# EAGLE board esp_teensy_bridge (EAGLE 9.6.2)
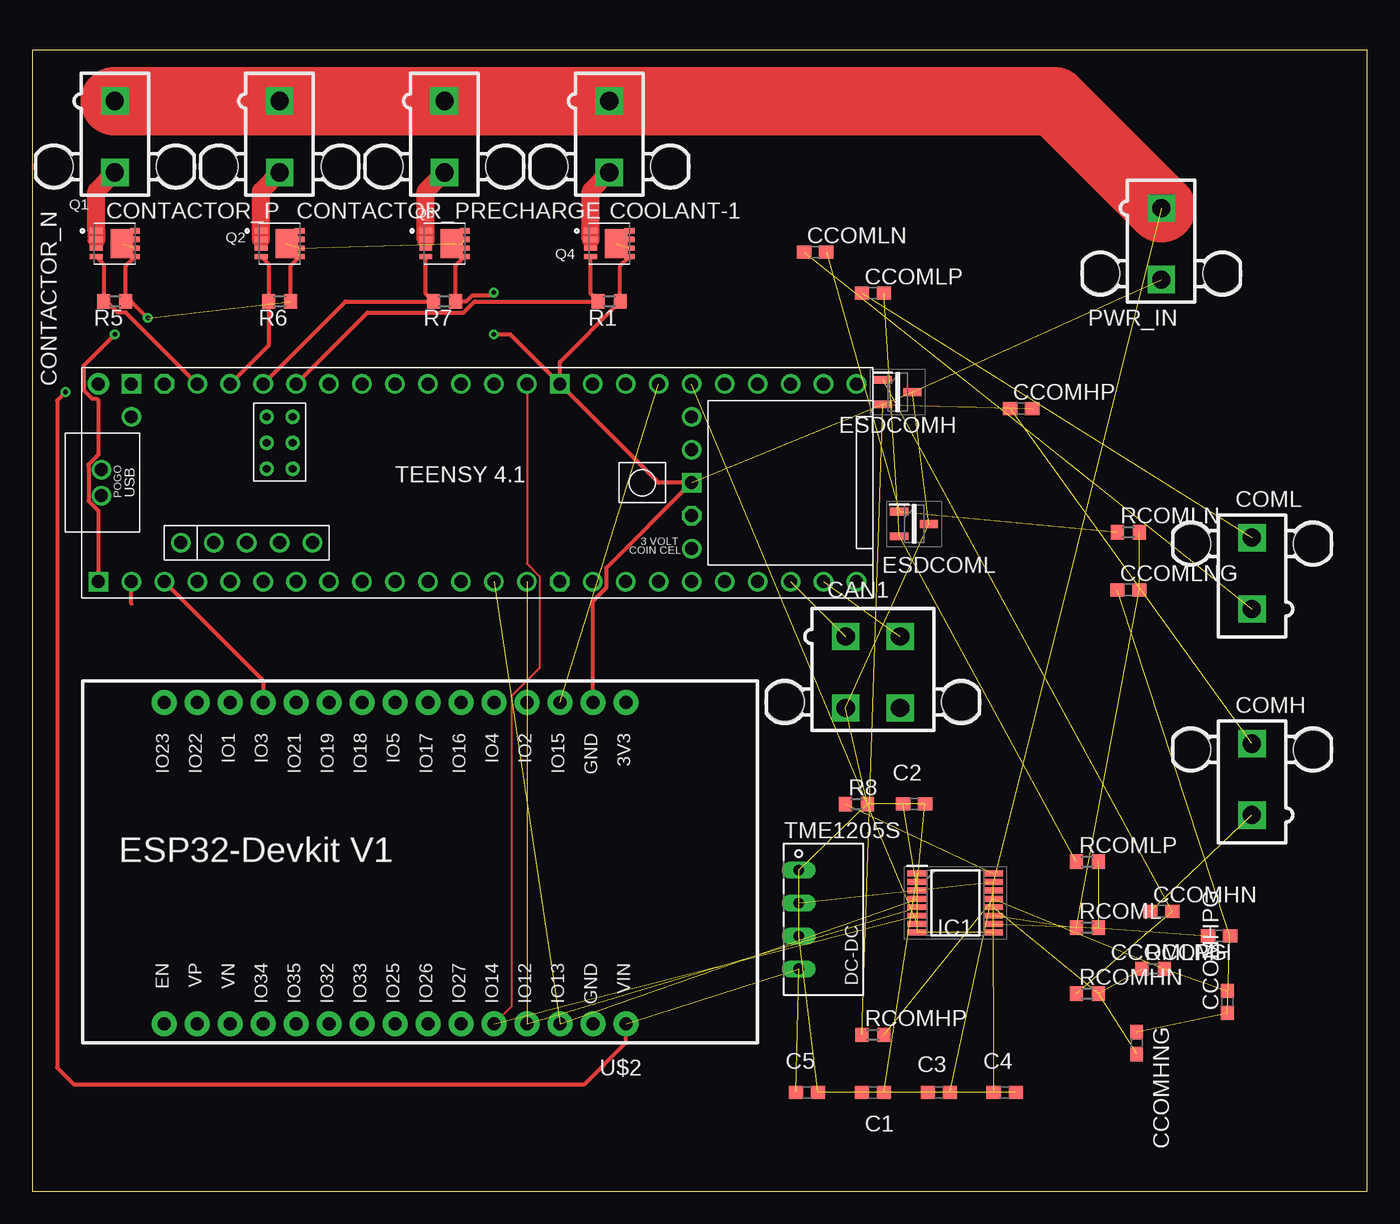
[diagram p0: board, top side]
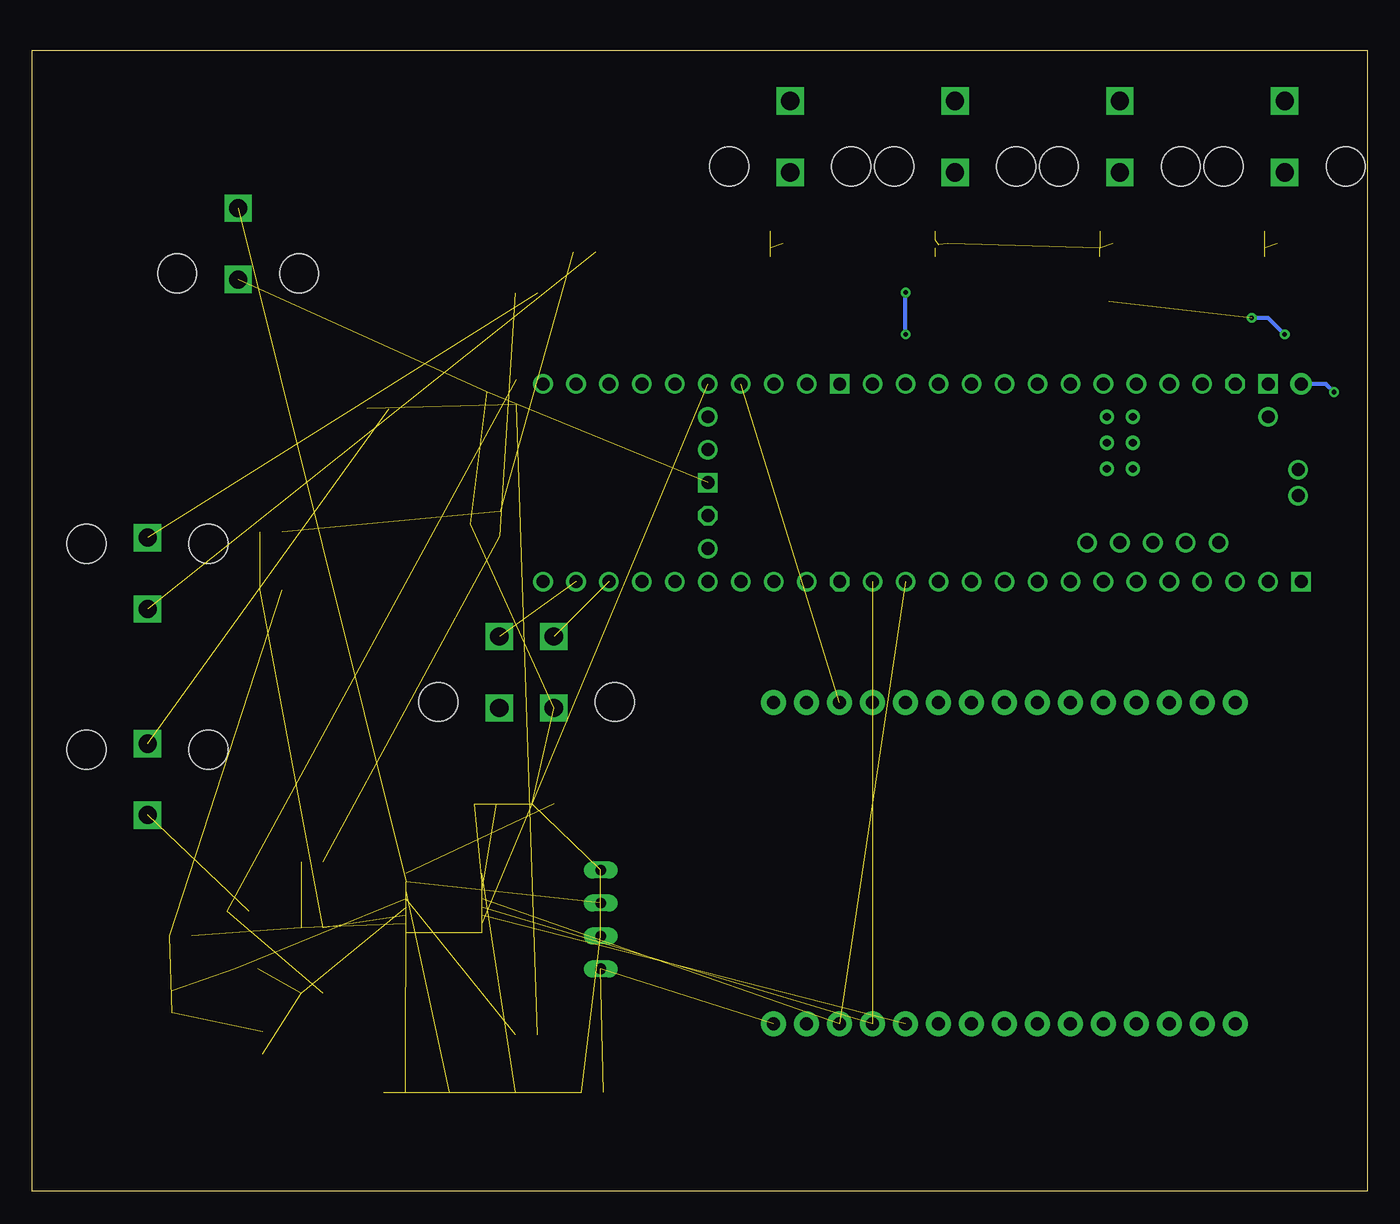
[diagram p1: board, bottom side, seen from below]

Size 102.85 x 87.94 mm. Coordinates in mm from the lower left corner, seen from the top.
Outline: 0,0 102.85,0 102.85,87.94 0,87.94 0,0
Copper layers (1*16): Top 0.035mm / dielectric 1.5mm / Bottom 0.035mm
Design rules "default": minimum track width 6mil, minimum drill 0.35mm, track to track 6mil, track to pad 6mil, pad to pad 6mil, via to via 6mil, smd to smd 6mil, copper to edge 40mil, drill to drill 6mil, minimum pad ring 10mil, minimum via ring 8mil, stop-mask expansion 4mil, vias tented up to drill 0mil, thermal gap 10mil

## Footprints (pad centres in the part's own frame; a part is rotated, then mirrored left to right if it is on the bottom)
C0603 = smd 1.1 x 1: 1 -0.85,0; 2 0.85,0
5566-4 = drill 1.4 square: 1 2.1,-2.75; 2 -2.1,-2.75; 3 2.1,2.75; 4 -2.1,2.75 | hole 3: 6.8,2.29; -6.8,2.29
5566-2 = drill 1.4 square: 1 0,-2.75; 2 0,2.75 | hole 3: 4.7,2.29; -4.7,2.29
SOT95P255X150-3N = smd 1.4 x 0.6: 1 -1.15,0.95; 2 -1.15,-0.95; 3 1.15,0
SOP65P640X120-16N = smd 1.475 x 0.45: 1 -2.938,2.275; 2 -2.938,1.625; 3 -2.938,0.975; 4 -2.938,0.325; 5 -2.938,-0.325; 6 -2.938,-0.975; 7 -2.938,-1.625; 8 -2.938,-2.275; 9 2.938,-2.275; 10 2.938,-1.625; 11 2.938,-0.975; 12 2.938,-0.325; 13 2.938,0.325; 14 2.938,0.975; 15 2.938,1.625; 16 2.938,2.275
VISHAY_SIS468DN-T1-GE3 = smd 0.99 x 0.405: 1 -1.435,0.99; 2 -1.435,0.33; 3 -1.435,-0.33; 4 -1.435,-0.99 | smd 0.76 x 0.405: 5 1.55,-0.99; 6 1.55,-0.33; 7 1.55,0.33; 8 1.55,0.99 | smd 1.725 x 2.235: 9 0.557,0
R0603 = smd 1 x 1.1: 1 -0.85,0; 2 0.85,0
NME = drill 0.813 long: 1 0,3.81; 2 0,1.27; 3 0,-1.27; 4 0,-3.81
ESP32-DEVKITV1 = drill 1 pad 1.93: 1 -22.87,-13.54; 2 -20.33,-13.54; 3 -17.79,-13.54; 4 -15.25,-13.54; 5 -12.71,-13.54; 6 -10.17,-13.54; 7 -7.63,-13.54; 8 -5.09,-13.54; 9 -2.55,-13.54; 10 -0.01,-13.54; 11 2.53,-13.54; 12 5.07,-13.54; 13 7.61,-13.54; 14 10.15,-13.54; 15 12.69,-13.54; 16 12.69,11.23; 17 10.15,11.23; 18 7.61,11.23; 19 5.07,11.23; 20 2.53,11.23; 21 -0.01,11.23; 22 -2.55,11.23; 23 -5.09,11.23; 24 -7.63,11.23; 25 -10.17,11.23; 26 -12.71,11.23; 27 -15.25,11.23; 28 -17.79,11.23; 29 -20.33,11.23; 30 -22.87,11.23
TEENSY41 = drill 1: 0-RX1/CS1/CRX2 -27.94,-7.62; 1-TX1/MISO1/CTX2 -25.4,-7.62; 2-OUT2 -22.86,-7.62; 3-LRCLK2 -20.32,-7.62; 4-BCLK2 -17.78,-7.62; 5-IN2 -15.24,-7.62; 6-OUT1D -12.7,-7.62; 7-RX2/OUT1A -10.16,-7.62; 8-TX2/IN1 -7.62,-7.62; 9-OUT1C -5.08,-7.62; 10-CS\MQSR -2.54,-7.62; 11-MOSI/CTX1 0,-7.62; 12-MISO/MQSL 2.54,-7.62; 13-SCK/LED 2.54,7.62; 14-A0/TX3/SPDIF_OUT 0,7.62; 15-A1/RX3/SPDIF_IN -2.54,7.62; 16-A2/RX4/SCL1 -5.08,7.62; 17-A3/TX4/SDA1 -7.62,7.62; 18-A4/SDA0 -10.16,7.62; 19-A5/SCL0 -12.7,7.62; 20-A6/TX5/LRCLK1 -15.24,7.62; 21-A7/RX5/BCLK1 -17.78,7.62; 22-A8/CTX1 -20.32,7.62; 23-A9/CRX1/MCLK1 -22.86,7.62; 24-A10/TX6/SCL2 7.62,-7.62; 25-A11/RX6/SDA2 10.16,-7.62; 26-A12/MOSI1 12.7,-7.62; 27-A13/SCK1 15.24,-7.62; 28-RX7 17.78,-7.62; 29-TX7 20.32,-7.62; 30-CRX3 22.86,-7.62; 31-CTX3 25.4,-7.62; 32-OUT1B 27.94,-7.62; 33-MCLK2 27.94,7.62; 34-RX8 25.4,7.62; 35-TX8 22.86,7.62; 36-PWM 20.32,7.62; 37-PWM 17.78,7.62; 38-A14/CS/IN1 15.24,7.62; 39-A15/CS/OUT1A 12.7,7.62; 40-A16/CS1 10.16,7.62; 41-A17/MISO1 7.62,7.62; +5V -24.13,-4.62; D+ -30.25,-1; D- -30.25,1; DM -21.59,-4.62; DP -19.05,-4.62; GND4 -16.51,-4.62; GND5 -13.97,-4.62; ON/OFF 15.24,5.08; PROGRAM 15.24,2.54; VBAT 15.24,-5.08; VUSB -27.94,5.08 | drill 1 octagon: 3V3-1 5.08,-7.62; 3V3-2 15.24,-2.54; 3V3-3 -25.4,7.62 | drill 0.6: G -15.51,3.08; LED -17.51,3.08; R+ -17.51,5.08; R- -15.51,5.08; T+ -15.51,1.08; T- -17.51,1.08 | drill 1 square: GND1 -30.48,-7.62; GND2 15.24,0; GND3 5.08,7.62; GND6 -27.94,7.62 | drill 1 pad 1.676: VIN -30.48,7.62

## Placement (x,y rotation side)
C1  0.22μF  [C0603]  64.77,7.62 180 top
C2  0.1μF  [C0603]  67.94,29.84 0 top
C3  0.22uF  [C0603]  69.85,7.62 0 top
C4  0.1μF  [C0603]  74.93,7.62 0 top
C5  0.22μF  [C0603]  59.69,7.62 0 top
CAN1  5566-4  [5566-4]  64.77,40.01 180 top
CCOMHN  2.2nf  [C0603]  87,21.59 0 top
CCOMHNG  220 pF  [C0603]  85.09,11.43 270 top
CCOMHP  2.2nf  [C0603]  76.2,60.33 0 top
CCOMHPG  220 pF  [C0603]  92.08,14.61 90 top
CCOMLN  2.2nf  [C0603]  60.33,72.39 0 top
CCOMLNG  220 pF  [C0603]  84.45,46.36 0 top
CCOMLP  2.2nf  [C0603]  64.77,69.22 0 top
CCOMLPG  220 pF  [C0603]  91.44,19.69 180 top
COMH  5566-2  [5566-2]  93.98,31.75 0 top
COML  5566-2  [5566-2]  93.98,47.62 0 top
CONTACTOR_N  5566-2  [5566-2]  6.35,81.28 180 top
CONTACTOR_P  5566-2  [5566-2]  19.05,81.28 180 top
CONTACTOR_PRECHARGE  5566-2  [5566-2]  31.75,81.28 180 top
COOLANT-1  5566-2  [5566-2]  44.45,81.28 180 top
ESDCOMH  ESDAVLC6-2BLY  [SOT95P255X150-3N]  66.67,61.59 0 top
ESDCOML  ESDAVLC6-2BLY  [SOT95P255X150-3N]  67.94,51.44 0 top
IC1  BQ79600PWRQ1  [SOP65P640X120-16N]  71.12,22.23 0 top
PWR_IN  5566-2  [5566-2]  87,73.03 180 top
Q1  SI7611DN-T1-GE3  [VISHAY_SIS468DN-T1-GE3]  6.35,73.03 0 top
Q2  SI7611DN-T1-GE3  [VISHAY_SIS468DN-T1-GE3]  19.05,73.03 0 top
Q3  SI7611DN-T1-GE3  [VISHAY_SIS468DN-T1-GE3]  31.75,73.03 0 top
Q4  SI7611DN-T1-GE3  [VISHAY_SIS468DN-T1-GE3]  44.45,73.03 0 top
R1  10k  [R0603]  44.45,68.58 180 top
R5  10k  [R0603]  6.35,68.58 180 top
R6  10k  [R0603]  19.05,68.58 180 top
R7  10k  [R0603]  31.75,68.58 180 top
R8  100k  [R0603]  63.5,29.84 0 top
RCOMH  1k  [R0603]  86.36,17.15 0 top
RCOMHN  49  [R0603]  81.28,15.24 0 top
RCOMHP  49  [R0603]  64.77,12.06 0 top
RCOML  1k  [R0603]  81.28,20.32 0 top
RCOMLN  49  [R0603]  84.45,50.8 0 top
RCOMLP  49  [R0603]  81.28,25.4 0 top
TME1205S  [NME]  59.05,20.96 0 top
U$2  ESP32DEVKITV1  [ESP32-DEVKITV1]  22.86,24.13 180 top
U$3  TEENSY41  [TEENSY41]  35.56,54.61 0 top

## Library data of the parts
C1-C5 CCOMHN CCOMHNG CCOMHP CCOMHPG CCOMLN CCOMLNG CCOMLP CCOMLPG = rcl; SPICEPREFIX: C
CAN1 = con-molex; MF: MOLEX; OC_FARNELL: unknown; OC_NEWARK: unknown
COMH COML CONTACTOR_N CONTACTOR_P CONTACTOR_PRECHARGE COOLANT-1 PWR_IN = con-molex; MF: MOLEX; OC_FARNELL: 1822072; OC_NEWARK: unknown
ESDCOMH ESDCOML = ESDAVLC6-2BLY; DESCRIPTION: STMICROELECTRONICS - ESDAVLC6-2BLY - ESD Protection Device, 17 V, SOT-23, 3 Pins, 5 V, 140 W, ESDA Transil Series; HEIGHT: 1.5mm; MANUFACTURER_NAME: STMicroelectronics; MANUFACTURER_PART_NUMBER: ESDAVLC6-2BLY; MOUSER_PART_NUMBER: 511-ESDAVLC6-2BLY; MOUSER_PRICE-STOCK: https://www.mouser.co.uk/ProductDetail/STMicroelectronics/ESDAVLC6-2BLY?qs=l7cgNqFNU1iH2e21evvYsA%3D%3D
IC1 = BQ79600; DESCRIPTION: Battery Management Automotive SPI/UART communication interface functional-safety compliant with automatic host wakeup; HEIGHT: 1.2mm; MANUFACTURER_NAME: Texas Instruments; MANUFACTURER_PART_NUMBER: BQ79600PWRQ1; MOUSER_PART_NUMBER: 595-BQ79600PWRQ1; MOUSER_PRICE-STOCK: https://www.mouser.co.uk/ProductDetail/Texas-Instruments/BQ79600PWRQ1?qs=bAKSY%2FctAC74v4PXQeVHrA%3D%3D
Q1-Q4 = SI7611DN-T1-GE3; AVAILABILITY: In Stock; DESCRIPTION: P-Channel 40 V 18A (Tc) 3.7W (Ta), 39W (Tc) Surface Mount PowerPAK® 1212-8; MF: Vishay Siliconix; MP: SI7611DN-T1-GE3; PACKAGE: PowerPAK®-1212 Vishay; PRICE: None; PURCHASE-URL: https://pricing.snapeda.com/search/part/SI7611DN-T1-GE3/?ref=eda
R1 R5-R8 RCOMH RCOMHN RCOMHP RCOML RCOMLN RCOMLP = rcl; SPICEPREFIX: R
TME1205S = dc-dc-converter; MF: C & D TECHNOLOGIES, INC; MPN: NME1205D; OC_FARNELL: 1021466; OC_NEWARK: 98B8198
U$2 = ESP32-DEVKITV1
U$3 = teensy

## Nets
5V: C5.1 TME1205S.4 U$2.30 U$3.VIN
COMHN: CCOMHNG.2 IC1.12 RCOMH.1 RCOMHN.2
COMHN_ISO: CCOMHN.1 COMH.1
COMHP: CCOMHPG.2 IC1.13 RCOMH.2 RCOMHP.2
COMHP_ISO: CCOMHP.1 COMH.2
COMLN: CCOMLNG.2 IC1.11 RCOML.1 RCOMLN.2
COMLN_ISO: CCOMLN.1 COML.1
COMLP: CCOMLPG.2 IC1.10 RCOML.2 RCOMLP.2
COMLP_ISO: CCOMLP.1 COML.2
CONTACTORN_CTRL: Q1.4 R5.2 U$3.23-A9/CRX1/MCLK1
CONTACTORP_CTRL: Q2.4 R6.2 U$3.22-A8/CTX1
CONTACTORPRECHARGE_CTRL: Q3.4 R7.2 U$3.21-A7/RX5/BCLK1
COOLANT_CTRL: Q4.4 R1.2 U$3.20-A6/TX5/LRCLK1
CS0: IC1.7 U$3.38-A14/CS/IN1
CS1: U$2.3 U$3.39-A15/CS/OUT1A
CS2: U$3.40-A16/CS1
GND: C1.2 C2.2 C3.1 C4.2 C5.2 CAN1.3 ESDCOMH.3 ESDCOML.3 IC1.2 IC1.8 IC1.9 PWR_IN.2 Q1.5 Q1.6 Q1.7 Q1.8 Q1.9 Q2.5 Q2.6 Q2.7 Q2.8 Q2.9 Q3.5 Q3.6 Q3.7 Q3.8 Q3.9 Q4.5 Q4.6 Q4.7 Q4.8 Q4.9 R1.1 R5.1 R6.1 R7.1 R8.2 TME1205S.1 TME1205S.3 U$2.2 U$3.GND1 U$3.GND2 U$3.GND3
GNDN: CCOMHNG.1 CCOMHPG.1 CCOMLNG.1 CCOMLPG.1
MISO: IC1.5 U$2.27 U$3.12-MISO/MQSL
MOSI: IC1.4 U$2.28 U$3.11-MOSI/CTX1
N$1: C1.1 IC1.1
N$2: CONTACTOR_P.2 Q2.1 Q2.2 Q2.3
N$3: C3.2 IC1.14
N$4: IC1.16 R8.1
N$5: CONTACTOR_N.2 Q1.1 Q1.2 Q1.3
N$6: COOLANT-1.2 Q4.1 Q4.2 Q4.3
N$7: CAN1.1 U$3.30-CRX3
N$8: CAN1.2 U$3.31-CTX3
N$10: CCOMLP.2 ESDCOML.2 RCOMLP.1
N$11: CCOMLN.2 ESDCOML.1 RCOMLN.1
N$12: CONTACTOR_PRECHARGE.2 Q3.1 Q3.2 Q3.3
N$15: CCOMHP.2 ESDCOMH.2 RCOMHP.1
N$16: CCOMHN.2 ESDCOMH.1 RCOMHN.1
NCS/CS: U$3.10-CS\MQSR
RX_BRIDGE: U$3.29-TX7
RX_ESP: U$3.1-TX1/MISO1/CTX2
SCK: IC1.6 U$2.26 U$3.13-SCK/LED
TX_BRIDGE: U$3.28-RX7
TX_ESP: U$3.0-RX1/CS1/CRX2
VCC: C4.1 CONTACTOR_N.1 CONTACTOR_P.1 CONTACTOR_PRECHARGE.1 COOLANT-1.1 IC1.15 PWR_IN.1 TME1205S.2
VIO: C2.1 IC1.3

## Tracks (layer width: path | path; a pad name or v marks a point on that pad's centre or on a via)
5V  (via drill 0.35)  (2 unrouted)
  Top 0.152: 45.72,11.43 45.73,11.44
  Top 0.305: v2.54,61.59 1.91,60.96 1.91,9.53 3.17,8.26 42.55,8.26 45.72,11.43 | 45.73,11.44 U$2.30
  Bottom 0.305: U$3.VIN 3.17,62.23 v2.54,61.59
COMHN  (3 unrouted)
COMHN_ISO  (1 unrouted)
COMHP  (3 unrouted)
COMHP_ISO  (1 unrouted)
COMLN  (3 unrouted)
COMLN_ISO  (1 unrouted)
COMLP  (3 unrouted)
COMLP_ISO  (1 unrouted)
CONTACTORN_CTRL
  Top 0.305: U$3.23-A9/CRX1/MCLK1 7.21,67.73 6.57,67.73 5.72,68.58 R5.2 5.5,71.45 Q1.4
CONTACTORP_CTRL
  Top 0.305: Q2.4 18.2,71.45 R6.2 18.2,65.19 U$3.22-A8/CTX1
CONTACTORPRECHARGE_CTRL
  Top 0.305: U$3.21-A7/RX5/BCLK1 24.13,68.58 R7.2 30.32,69.17 Q3.4
COOLANT_CTRL
  Top 0.305: U$3.20-A6/TX5/LRCLK1 25.82,67.73 33.23,67.73 34.08,68.58 R1.2 43.02,69.17 Q4.4
CS0  (1 unrouted)
CS1  (1 unrouted)
GND  (via drill 0.35)  (33 unrouted)
  Top 0.152: 4.95,56.64 5.08,56.77 | 4.33,55.88 4.33,56.02 | Q3.6 33.03,72.97
  Top 0.305: 5.08,56.77 5.08,60.96 4.95,61.09 4.61,61.09 3.94,61.76 3.94,63.63 v6.35,66.04 | 4.95,56.64 4.33,56.02 | 4.33,55.88 4.33,53.2 5.08,52.45 U$3.GND1 | v8.89,67.31 7.62,68.58 R5.1 7.2,71.34 Q1.5 | R6.1 19.9,71.34 Q2.5 | Q3.5 32.6,71.34 R7.1 33.43,68.58 33.89,69.04 35.33,69.04 v35.56,69.26 | U$3.GND3 36.83,66.04 v35.56,66.04 | U$3.GND3 40.64,63.92 R1.1 45.3,71.34 Q4.5 | U$3.GND3 48.26,54.61 U$3.GND2 44.24,48.05 44.24,46.55 43.19,45.5 U$2.2
  Bottom 0.305: v6.35,66.04 7.62,67.31 v8.89,67.31 | v35.56,66.04 v35.56,69.26
GNDN  (3 unrouted)
MISO  (2 unrouted)
MOSI  (2 unrouted)
N$1  (1 unrouted)
N$2
  Top 0.152: Q2.2 Q2.3
  Top 1.372: Q2.2 Q2.1 17.61,77.09 CONTACTOR_P.2
N$3  (1 unrouted)
N$4  (1 unrouted)
N$5
  Top 0.152: Q1.3 Q1.2
  Top 1.372: Q1.2 Q1.1 4.92,77.09 CONTACTOR_N.2
N$6
  Top 0.152: Q4.3 Q4.2
  Top 1.372: Q4.2 Q4.1 43.02,77.09 COOLANT-1.2
N$7  (1 unrouted)
N$8  (1 unrouted)
N$10  (2 unrouted)
N$11  (2 unrouted)
N$12
  Top 0.152: Q3.3 Q3.2
  Top 1.372: Q3.2 Q3.1 30.32,77.09 CONTACTOR_PRECHARGE.2
N$15  (2 unrouted)
N$16  (2 unrouted)
RX_ESP
  Top 0.305: U$3.1-TX1/MISO1/CTX2 17.79,39.36 17.79,38.1
SCK  (1 unrouted)
  Top 0.152: U$3.13-SCK/LED 38.1,48.38 39.08,47.4 39.08,40.33 36.92,38.16 36.92,14.25 U$2.26
TX_ESP
  Top 0.305: 7.62,45.3 U$3.0-RX1/CS1/CRX2
VCC  (3 unrouted)
  Top 5.283: CONTACTOR_N.1 CONTACTOR_P.1 CONTACTOR_PRECHARGE.1 COOLANT-1.1 78.74,84.03 PWR_IN.1
VIO  (1 unrouted)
